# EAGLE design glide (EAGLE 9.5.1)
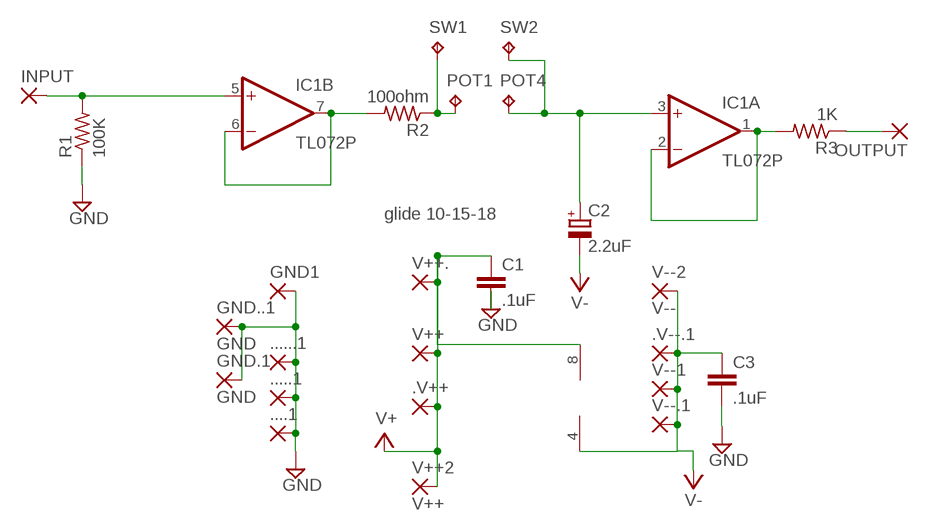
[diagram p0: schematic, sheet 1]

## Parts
....1  3,17/1,3  [3,17/1,3]
.....1  3,17/1,3  [3,17/1,3]
......1  3,17/1,3  [3,17/1,3]
.V++  2,54/1,0  [2,54/1,0]
.V--.1  3,17/1,3  [3,17/1,3]
C1  .1uF  C5/2.5  [C5B2.5]
C2  2.2uF  CPOL-EUE3.5-10  [E3,5-10]
C3  .1uF  C5/2.5  [C5B2.5]
GND1  3,17/1,3  [3,17/1,3]
GND.1  GND  1,6/0,8  [1,6/0,8]
GND..1  GND  1,6/0,8  [1,6/0,8]
IC1  TL072P  [DIL08]
INPUT  3,17/1,3  [3,17/1,3]
OUTPUT  3,17/1,3  [3,17/1,3]
POT1  TPPAD1-17Y  [P1-17Y]
POT4  TPPAD1-17Y  [P1-17Y]
R1  100K  R-US_0204/7  [0204/7]
R2  100ohm  R-US_0204/7  [0204/7]
R3  1K  R-US_0204/7  [0204/7]
SW1  TPPAD1-17Y  [P1-17Y]
SW2  TPPAD1-17Y  [P1-17Y]
V++  2,54/1,0  [2,54/1,0]
V++2  V++  1,6/0,8  [1,6/0,8]
V++.  2,54/1,0  [2,54/1,0]
V--1  3,17/1,3  [3,17/1,3]
V--2  V--  1,6/0,8  [1,6/0,8]
V--.1  3,17/1,3  [3,17/1,3]

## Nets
GND: ....1.1(P) .....1.1(P) ......1.1(P) C1.2 C3.2 GND1.1(P) GND.1.1(P) GND..1.1(P) R1.1
N$1: IC1.5(B:+IN) INPUT.1(P) R1.2
N$2: IC1.6(B:-IN) IC1.7(B:OUT) R2.2
N$3: IC1.1(A:OUT) IC1.2(A:-IN) R3.2
N$4: OUTPUT.1(P) R3.1
N$5: POT1.TP R2.1 SW1.TP
N$6: C2.+ IC1.3(A:+IN) POT4.TP SW2.TP
V+: .V++.1(P) C1.1 IC1.8(P:V+) V++2.1(P) V++.1(P) V++..1(P)
V-: .V--.1.1(P) C2.- C3.1 IC1.4(P:V-) V--1.1(P) V--2.1(P) V--.1.1(P)

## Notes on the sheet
- glide 10-15-18

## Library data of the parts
....1 .....1 ......1 GND1 INPUT OUTPUT = wirepad:3,17/1,3: THROUGH-HOLE PAD
.V++ V++ V++. = wirepad-NONAMES:2,54/1,0: THROUGH-HOLE PAD
.V--.1 V--1 V--.1 = wirepad-NONAMES:3,17/1,3: THROUGH-HOLE PAD
C1 C3 = capacitor-wima:C: CAPACITOR
C2 = rcl:CPOL-EU: POLARIZED CAPACITOR, European symbol; SPICEPREFIX: C
GND.1 GND..1 V++2 V--2 = wirepad-NONAMES:1,6/0,8: THROUGH-HOLE PAD
IC1 = linear:TL072: OP AMP
POT1 POT4 SW1 SW2 = testpad:TP: Test pad
R1-R3 = rcl:R-US_: RESISTOR, American symbol

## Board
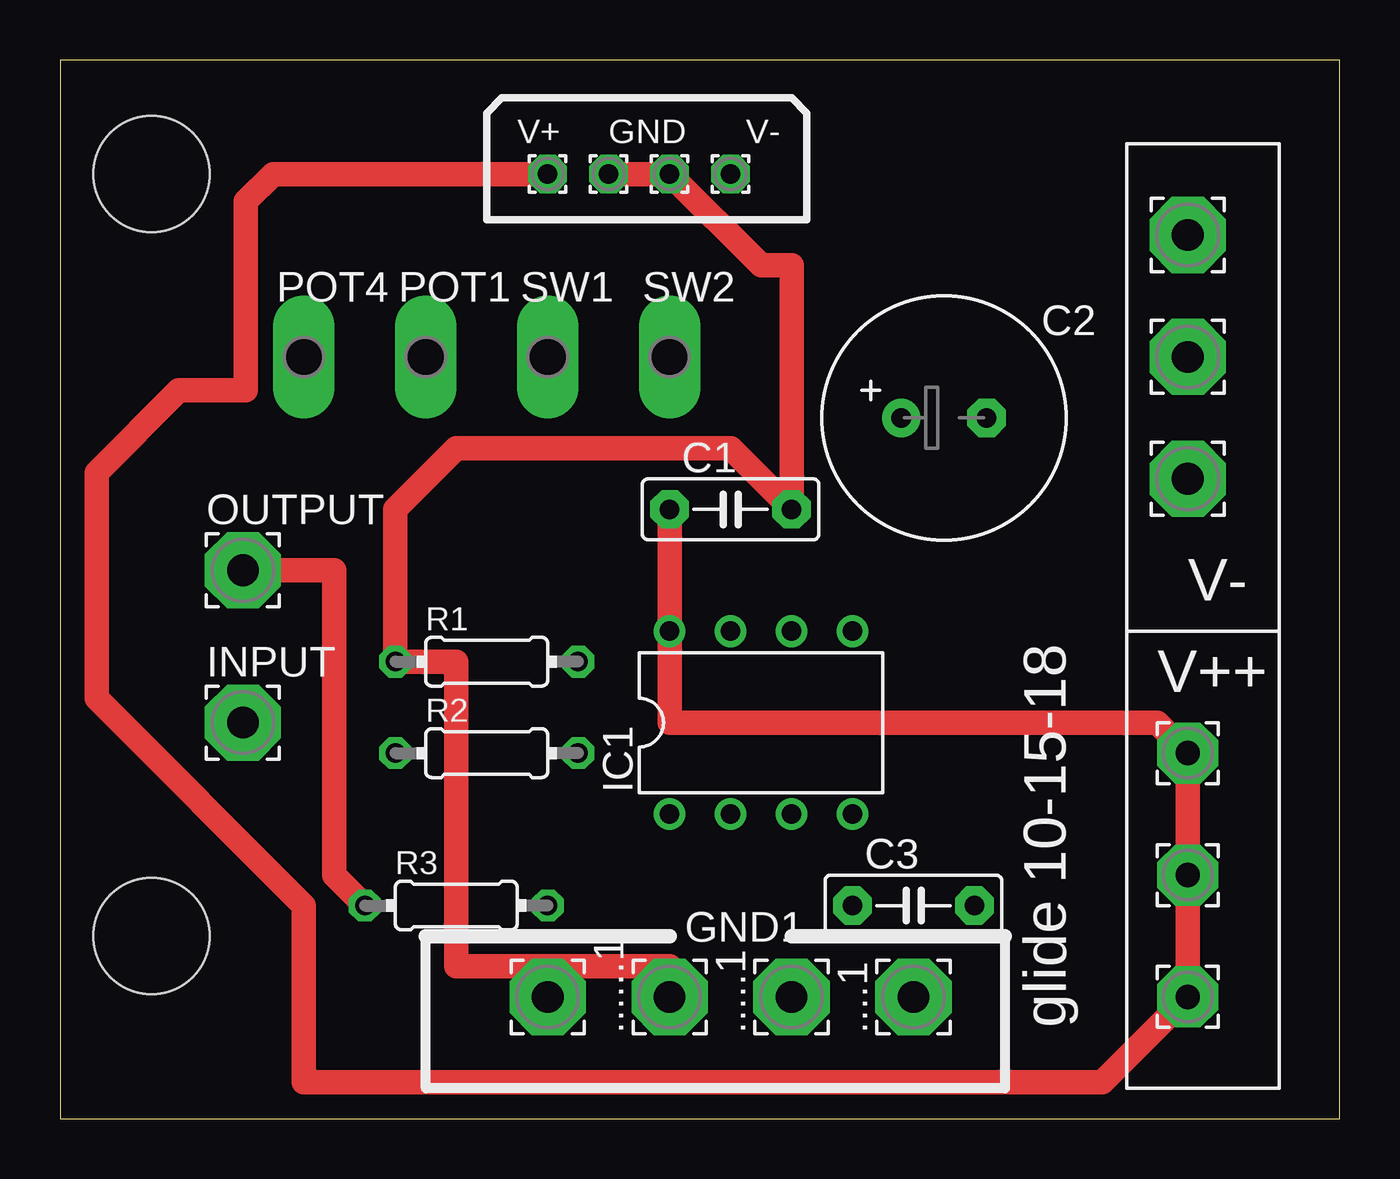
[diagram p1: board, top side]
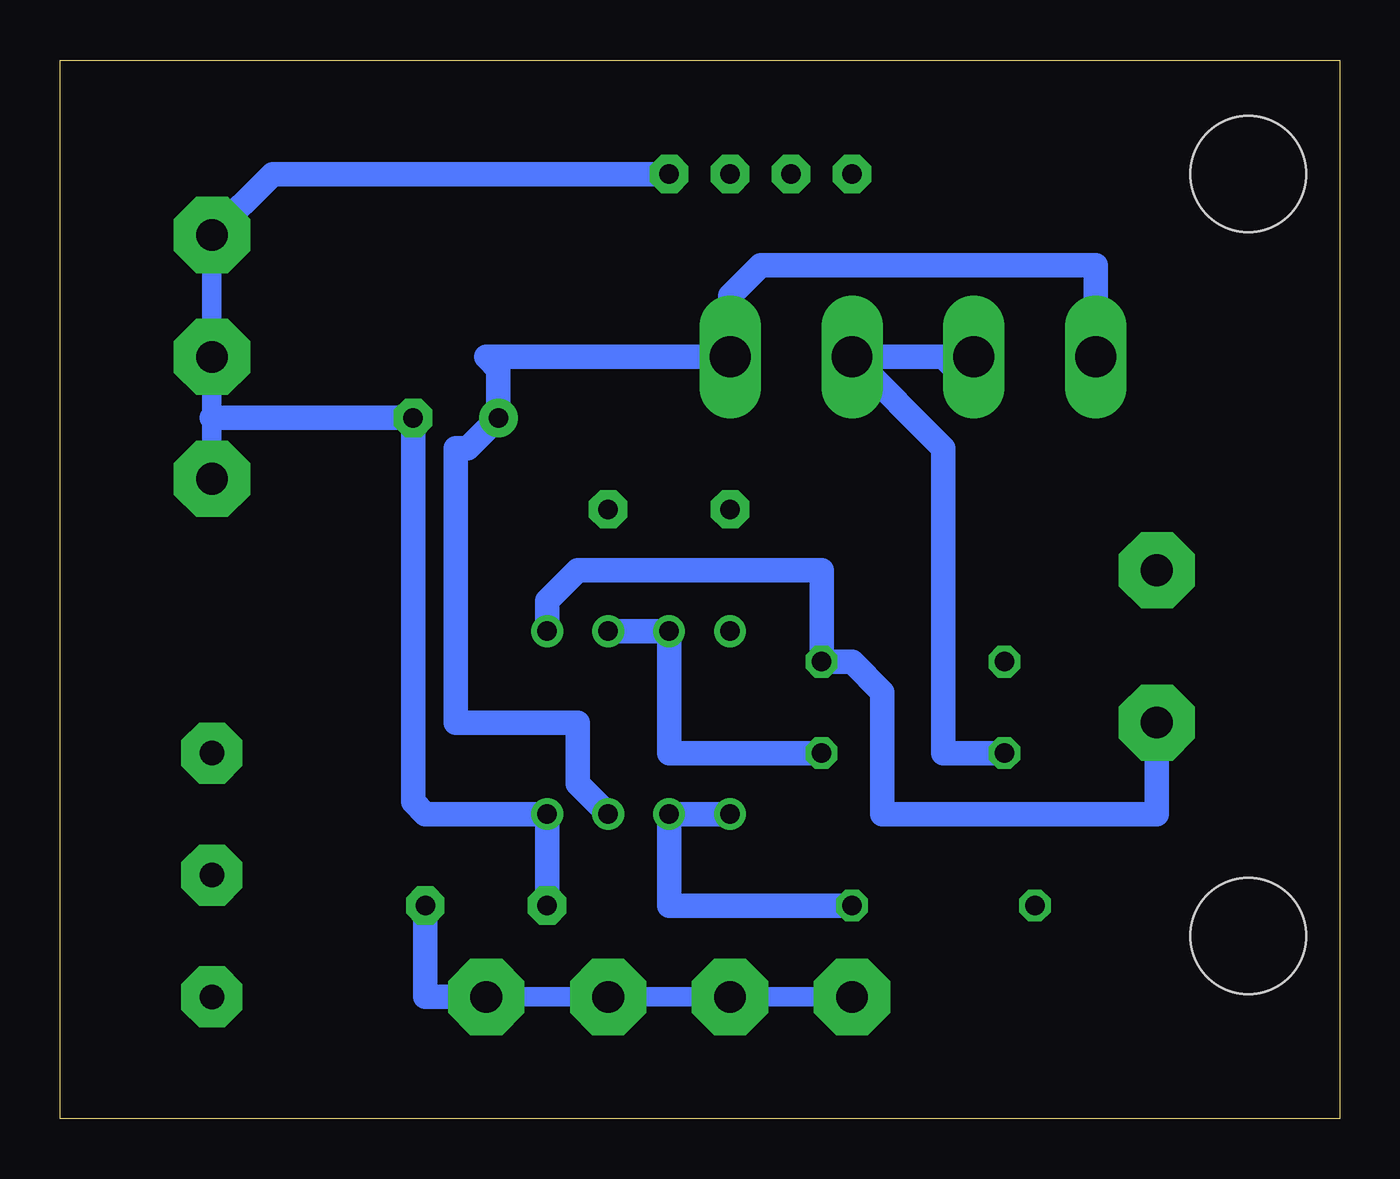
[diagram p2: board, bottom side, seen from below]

Size 53.32 x 44.12 mm. Coordinates in mm from the lower left corner, seen from the top.
Outline: 0,0 53.32,0 53.32,44.12 0,44.12 0,0
Copper layers (1*16): Top 0.035mm / dielectric 1.5mm / Bottom 0.035mm
Design rules "default": minimum track width 6mil, minimum drill 0.35mm, track to track 6mil, track to pad 6mil, pad to pad 6mil, via to via 6mil, smd to smd 6mil, copper to edge 40mil, drill to drill 6mil, minimum pad ring 10mil, minimum via ring 8mil, stop-mask expansion 4mil, vias tented up to drill 0mil, thermal gap 10mil
Holes 4.83 mm at 3.81,39.37 3.81,7.62

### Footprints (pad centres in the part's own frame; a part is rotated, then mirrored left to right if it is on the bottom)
3,17/1,3 = drill 1.321 pad 3.175 octagon: 1 0,0
2,54/1,0 = drill 1.016 pad 2.54 octagon: 1 0,0
C5B2.5 = drill 0.813 pad 1.6 octagon: 1 -2.54,0; 2 2.54,0
E3,5-10 = drill 0.813 pad 1.6: + -1.778,0 | drill 0.813 pad 1.6 octagon: - 1.778,0
1,6/0,8 = drill 0.813 pad 1.6 octagon: 1 0,0
DIL08 = drill 0.813 pad 1.27: 1 -3.81,-3.81; 2 -1.27,-3.81; 3 1.27,-3.81; 4 3.81,-3.81; 5 3.81,3.81; 6 1.27,3.81; 7 -1.27,3.81; 8 -3.81,3.81
P1-17Y = drill 1.702 pad 2.121 long: TP 0,0
0204/7 = drill 0.813 octagon: 1 -3.81,0; 2 3.81,0

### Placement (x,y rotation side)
....1  35.56,5.08 90 top
.....1  30.48,5.08 90 top
......1  25.4,5.08 90 top
.V++  46.99,15.24 0 top
.V--.1  46.99,26.67 0 top
C1  27.94,25.4 0 top
C2  36.83,29.21 0 top
C3  35.56,8.89 0 top
GND1  20.32,5.08 90 top
GND.1  25.4,39.37 0 top
GND..1  22.86,39.37 0 top
IC1  29.21,16.51 0 top
INPUT  7.62,16.51 0 top
OUTPUT  7.62,22.86 0 top
POT1  15.24,31.75 0 top
POT4  10.16,31.75 0 top
R1  17.78,19.05 0 top
R2  17.78,15.24 0 top
R3  16.51,8.89 0 top
SW1  20.32,31.75 0 top
SW2  25.4,31.75 0 top
V++  46.99,10.16 0 top
V++2  20.32,39.37 0 top
V++.  46.99,5.08 0 top
V--1  46.99,31.75 0 top
V--2  27.94,39.37 0 top
V--.1  46.99,36.83 0 top

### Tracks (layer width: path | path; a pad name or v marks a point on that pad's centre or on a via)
GND
  Top 1.016: ......1.1 25.4,6.35 16.51,6.35 16.51,19.05 R1.1 13.97,25.4 16.51,27.94 27.94,27.94 C1.2 30.48,35.56 29.21,35.56 GND.1.1 GND..1.1
  Bottom 0.813: ....1.1 .....1.1 ......1.1 GND1.1
  Bottom 1.016: ....1.1 38.1,5.08 C3.2
N$1
  Bottom 1.016: IC1.5 33.02,21.59 31.75,22.86 21.59,22.86 R1.2 20.32,19.05 19.05,17.78 19.05,12.7 7.62,12.7 INPUT.1
N$2
  Bottom 1.016: R2.2 27.94,15.24 IC1.7 IC1.6
N$3
  Bottom 1.016: R3.2 27.94,8.89 IC1.2 IC1.1
N$4
  Top 1.016: R3.1 11.43,10.16 11.43,22.86 OUTPUT.1
N$5
  Bottom 1.016: R2.1 16.51,15.24 16.51,27.94 SW1.TP 16.51,31.75 15.24,30.48 POT1.TP
N$6
  Bottom 1.016: IC1.3 31.75,13.97 31.75,16.51 36.83,16.51 36.83,27.94 36.32,27.94 C2.+ 35.05,31.24 35.56,31.75 SW2.TP 25.4,34.29 24.13,35.56 10.16,35.56 POT4.TP
V+
  Top 1.016: V++2.1 8.89,39.37 7.75,38.23 7.75,30.35 4.95,30.35 1.52,26.92 1.52,17.53 10.16,8.89 10.16,1.52 43.43,1.52 V++..1 V++.1 .V++.1 45.72,16.51 25.4,16.51 IC1.8 C1.1
V-
  Bottom 0.813: V--.1.1 V--1.1 46.99,29.21 .V--.1.1
  Bottom 1.016: C3.1 IC1.4 38.1,12.7 38.61,13.21 C2.- 46.99,29.21 | V--.1.1 44.45,39.37 V--2.1

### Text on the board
tNames: V+ | GND | V- | V- | V++ | glide 10-15-18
